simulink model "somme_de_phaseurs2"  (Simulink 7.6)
settings: Solver=ode23tb  StartTime=0.0  StopTime=0.02  RelTol=1e-3
InitFcn:
  | clc, close all
StopFcn:
  | close all
  | load somme_2_sinusoïdes.mat
  | plot(x(1,:),x(2,:))
  | gtext('5 sin wt')
  | pause(10)
  | hold on
  | plot(x(1,:),x(3,:))
  | gtext('')
  | pause(10)
  | hold on
  | plot(x(1,:),x(4,:))
  | gtext('')
  | pause(10)
  | hold on
  | plot(x(1,:),x(5,:))
  | gtext('')
  | pause(10)
  | hold on
  | grid
  | title('Somme instantanée de 2 sinusoïdes')
  | xlabel('temps')
libraries: powerlib x11

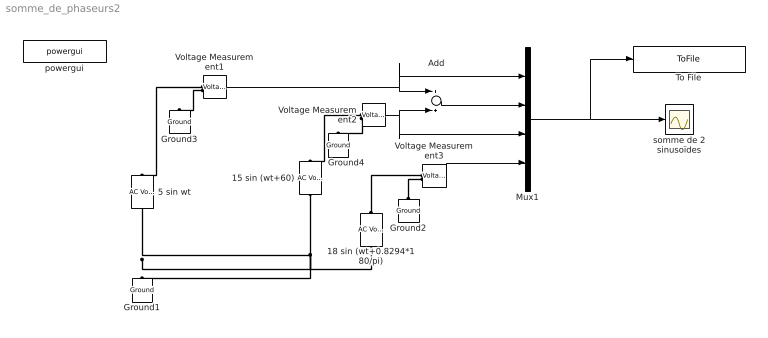
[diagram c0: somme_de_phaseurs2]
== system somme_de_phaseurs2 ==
  15 sin (wt+60) : powerlib/Electrical Sources/AC Voltage Source  DialogController=POWERSYS.PowerSysDialog  SystemSampleTime=-1  Amplitude=15  Phase=60  Frequency=60  SampleTime=0  Measurements=None
  18 sin (wt+0.8294*180/pi) : powerlib/Electrical Sources/AC Voltage Source  DialogController=POWERSYS.PowerSysDialog  SystemSampleTime=-1  Amplitude=18  Phase=0.8294*180/pi  Frequency=60  SampleTime=0  Measurements=None
  5 sin wt : powerlib/Electrical Sources/AC Voltage Source  DialogController=POWERSYS.PowerSysDialog  SystemSampleTime=-1  Amplitude=5  Phase=0  Frequency=60  SampleTime=0  Measurements=None
  Add : Sum
  Ground{1..4} (4 alike) : powerlib/Elements/Ground  DialogController=POWERSYS.PowerSysDialog  PhysicalDomain=powersysdomain  SubClassName=unknown  LeftPortType=p1  RightPortType=p1  LConnTagsString=a
  Mux1 : Mux
  To File : ToFile  Filename=somme_2_sinusoïdes  MatrixName=x
  Voltage Measurement1 : powerlib/Measurements/Voltage Measurement  DialogController=POWERSYS.PowerSysDialog  SystemSampleTime=-1  PhasorSimulation=off  OutputType=Complex  PSBequivalent=0
  Voltage Measurement2 : powerlib/Measurements/Voltage Measurement  DialogController=POWERSYS.PowerSysDialog  SystemSampleTime=-1  PhasorSimulation=off  OutputType=Complex  PSBequivalent=0
  Voltage Measurement3 : powerlib/Measurements/Voltage Measurement  DialogController=POWERSYS.PowerSysDialog  SystemSampleTime=-1  PhasorSimulation=off  OutputType=Complex  PSBequivalent=0
  powergui : powerlib/powergui  SystemSampleTime=-1  SimulationMode=Continuous  SampleTime=0  frequency=60  SPID=off  DisableSnubberDevices=off  DisableRonSwitches=off  DisableVfSwitches=off  SwTol=0  Interpol=off  frequencyindice=60  echomessages=off  HookPort=off  DisplayEquations=off  FunctionMessages=off  EnableUseOfTLC=off  x0status=blocks  RestoreLinks=warning  ResistiveCurrentMeasurement=off  Frange=[0:2:500]  Ylog=off  Xlog=on  ShowGrid=off  save=off  variable=ZData  ZoomFFT=on  StartTime=0.0  cycles=1  DisplayStyle=1  fundamental=60  FreqAxis=off  MaxFrequency=1000  frequencyindicesteady=1  RmsSteady=1  display=off  Ts=0  methode=off
  somme de 2 sinusoïdes : Scope
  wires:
  Voltage Measurement2/1 -> Add/2, Mux1/3
  Voltage Measurement1/1 -> Add/1, Mux1/1
  Add/1 -> Mux1/2
  Mux1/1 -> somme de 2 sinusoïdes/1, To File/1
  Voltage Measurement3/1 -> Mux1/4
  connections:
  Voltage Measurement1/LConn1 -- 5 sin wt/RConn1
  Voltage Measurement1/LConn2 -- Ground3/LConn1
  Voltage Measurement2/LConn1 -- 15 sin (wt+60)/RConn1
  5 sin wt/LConn1 -- Ground1/LConn1 -- 15 sin (wt+60)/LConn1 -- 18 sin (wt+0.8294*180/pi)/LConn1
  Voltage Measurement2/LConn2 -- Ground4/LConn1
  18 sin (wt+0.8294*180/pi)/RConn1 -- Voltage Measurement3/LConn1
  Ground2/LConn1 -- Voltage Measurement3/LConn2
